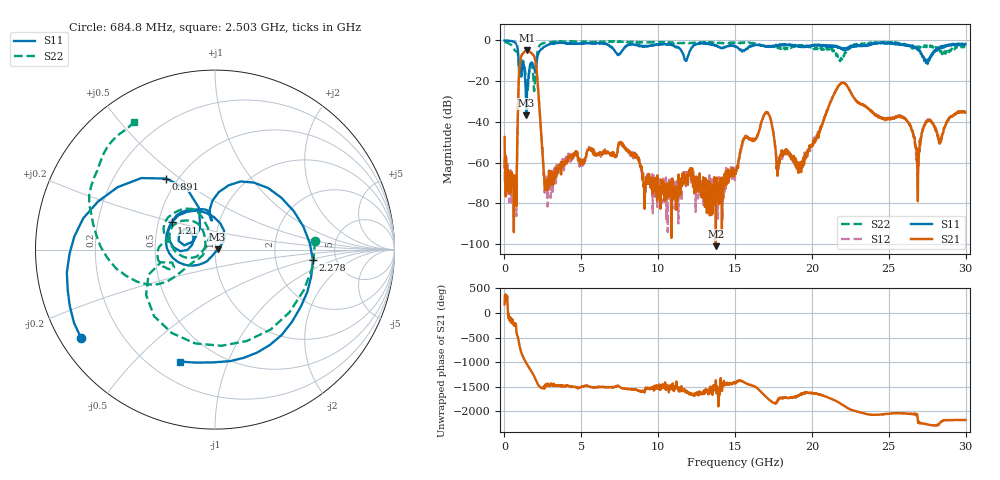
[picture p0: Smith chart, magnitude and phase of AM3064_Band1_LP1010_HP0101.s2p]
# Hz S DB R 50.0
!freq dBS11 angS11 dBS21 angS21 dBS12 angS12 dBS22 angS22
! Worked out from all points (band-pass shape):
!   1600 points, 10 MHz to 29.98 GHz, reference 50 ohm
!   highest |S21| = -4.95 dB at 1.453 GHz (marker M1); lowest = -101.0 dB at 13.75 GHz (marker M2)
!   |S21| within 3 dB of the highest: 1.084 GHz to 1.929 GHz (845 MHz wide, 56.1 % of centre)
!   lowest |S11| = -36.7 dB at 1.416 GHz (marker M3), VSWR 1.03, Z = 51.5 + j0.124 ohm
!   |S11| at or under -10 dB: 916.8 MHz to 2.107 GHz (1.191 GHz wide, 78.7 % of centre); 27.39325 GHz to 27.45994 GHz (66.69 MHz wide, 0.243 % of centre); 27.49016 GHz to 27.56382 GHz (73.67 MHz wide, 0.268 % of centre)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
!   |S22| runs from -24.9 to -0.4 dB; largest |S21 - S12| = 0.007
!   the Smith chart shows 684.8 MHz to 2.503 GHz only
!   S11 on the Smith chart (normalised r, x): 684.8 MHz: 0.06, -0.30; 891 MHz: 0.43, +0.45; 1.21 GHz: 0.59, +0.19; 2.278 GHz: 3.33, -0.55; 2.503 GHz: 0.31, -0.69
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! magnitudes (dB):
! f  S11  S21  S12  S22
! 10 MHz  0.0  -47.4  -58.1  -0.4
! 684.8 MHz  -1.0  -68.1  -66.8  -5.1
! 891 MHz  -6.4  -29.9  -29.9  -8.0
! 1.21 GHz  -10.9  -6.4  -6.3  -10.0
! 1.416 GHz  -36.7  -5.0  -4.9  -20.8
! 1.453 GHz  -26.8  -5.0  -4.9  -22.4
! 1.959 GHz  -14.2  -8.6  -8.5  -22.4
! 2.278 GHz  -5.2  -33.3  -33.3  -2.6
! 2.503 GHz  -3.7  -58.0  -60.4  -1.5
! 5.015 GHz  -1.4  -59.3  -60.2  -0.8
! 7.564 GHz  -6.2  -50.4  -50.4  -0.5
! 10 GHz  -2.0  -72.5  -75.2  -1.0
! 13.75 GHz  -2.5  -101.0  -72.4  -1.2
! 15 GHz  -2.9  -64.2  -64.5  -1.4
! 17.03 GHz  -3.0  -35.2  -35.3  -3.2
! 17.8 GHz  -2.2  -61.5  -61.8  -3.5
! 19.99 GHz  -2.9  -51.4  -51.6  -3.2
! 21.94 GHz  -4.1  -20.8  -20.8  -9.4
! 25 GHz  -1.1  -38.7  -38.0  -1.0
! 26.87 GHz  -4.3  -68.2  -71.2  -3.1
! 27.49 GHz  -9.9  -39.5  -39.1  -3.1
! 29.98 GHz  -1.8  -35.4  -35.0  -3.1
